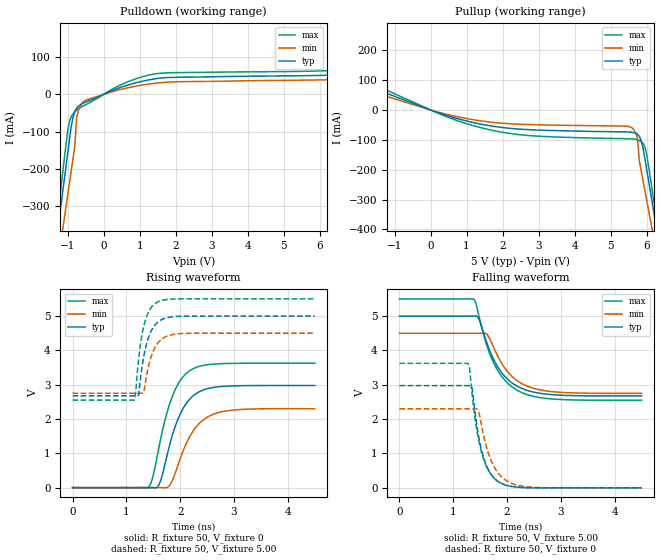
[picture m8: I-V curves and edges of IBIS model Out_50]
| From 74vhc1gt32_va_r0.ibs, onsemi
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|//////////////////////////////////////////////////////////////////////////////
|//////////////////////////////////////////////////////////////////////////////
[Model] Out_50
Model_type Output
Polarity Non-Inverting
Vmeas = 2.50
Vref = 5.00
Rref = 1k
Cref = 15pF
|  variable   typ   min   max
C_comp   3.9pF   3.9pF   3.9pF
|//////////////////////////////////////////////////////////////////////////////
[Temperature Range]   25   125   -55
|//////////////////////////////////////////////////////////////////////////////
[Voltage Range]   5.00V   4.50V   5.50V
|//////////////////////////////////////////////////////////////////////////////
[Pulldown Reference]   0V   0V   0V
|//////////////////////////////////////////////////////////////////////////////
[Pullup Reference]   5.00V   4.50V   5.50V
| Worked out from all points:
|   slope of the pulldown table from 0 to 0.75 V, typ, clamps not added: 27.5 ohm
|   slope of the pullup table from 0 to 0.75 V, typ, clamps not added: 25.7 ohm
|   falling waveform, R_fixture 50, V_fixture 5.00: 20-80 % time 466ps typ, 472ps min, 463ps max; typ from 5 V to 2.67 V
|   falling waveform, R_fixture 50, V_fixture 0: 20-80 % time 239ps typ, 298ps min, 250ps max; typ from 2.98 V to 0 V
|   rising waveform, R_fixture 50, V_fixture 0: 20-80 % time 378ps typ, 421ps min, 372ps max; typ from 0 V to 2.98 V
|   rising waveform, R_fixture 50, V_fixture 5.00: 20-80 % time 192ps typ, 200ps min, 168ps max; typ from 2.67 V to 5 V
|//////////////////////////////////////////////////////////////////////////////
[Pulldown]
|   Voltage   I(typ)   I(min)   I(max)
-5V       -3.203A    -2.93A     -3.469A
-1.4V     -459.9mA   -538mA     -431.9mA
-1.25V    -347.3mA   -438.3mA   -305.4mA
-1.15V    -272.2mA   -371.8mA   -221.3mA
-950mV    -121.9mA   -238.6mA   -72.82mA
-850mV    -61mA      -171.9mA   -52.46mA
-750mV    -36.79mA   -62.89mA   -42.39mA
-700mV    -31.75mA   -43.7mA    -38.5mA
125mV     5.571mA    3.909mA    7.607mA
1.5V      42.83mA    30.68mA    56.15mA
8V        63.99mA    47.99mA    80.81mA
10V       113.3mA    83.22mA    177.5mA
|//////////////////////////////////////////////////////////////////////////////
[Pullup]
|   Voltage   I(typ)   I(min)   I(max)
-5V       205mA      169.6mA    275.2mA
-3.8V     161.9mA    134.7mA    191.7mA
1.15V     -41.19mA   -31.93mA   -51.29mA
5.55V     -74.1mA    -57.09mA   -96.6mA
5.75V     -81.39mA   -96.38mA   -99.99mA
5.8V      -88.37mA   -170.9mA   -102.6mA
5.85V     -102.5mA   -203.1mA   -106mA
6V        -196.5mA   -299.9mA   -146.2mA
6.15V     -305mA     -396.6mA   -263.3mA
6.25V     -377.3mA   -461.2mA   -343.4mA
6.4V      -485.9mA   -558mA     -463.7mA
10V       -3.241A    -3.004A    -3.527A
|//////////////////////////////////////////////////////////////////////////////
|//////////////////////////////////////////////////////////////////////////////
[Ramp]
|  variable   typ   min   max
dV/dt_f   1.395E+00/4.500E-10  1.050E+00/4.750E-10  1.770E+00/4.750E-10
dV/dt_r   1.785E+00/3.750E-10  1.380E+00/4.250E-10  2.175E+00/3.750E-10
R_load = 50
|/////////////////////////////////////////////////////////////////////////////
[Falling Waveform]
R_fixture = 50
V_fixture = 5.00
V_fixture_min = 4.50
V_fixture_max = 5.50
C_fixture = 0p
|   time   V(typ)   V(min)   V(max)
0s        5V         4.5V       5.5V
1.375ns   5.001V     4.5V       5.5V
1.425ns   5.001V     4.5V       5.343V
1.475ns   4.921V     4.5V       5.016V
1.625ns   4.214V     4.472V     4.138V
1.775ns   3.661V     4V         3.561V
2ns       3.175V     3.398V     3.064V
2.275ns   2.893V     3.032V     2.773V
2.9ns     2.706V     2.792V     2.58V
4.5ns     2.675V     2.75V      2.55V
|//////////////////////////////////////////////////////////////////////////////
[Falling Waveform]
R_fixture = 50
V_fixture = 0
C_fixture = 0p
|   time   V(typ)   V(min)   V(max)
0s        2.975V     2.3V       3.625V
1.275ns   2.975V     2.3V       3.624V
1.3ns     2.975V     2.3V       3.522V
1.35ns    2.905V     2.3V       2.73V
1.45ns    1.698V     2.287V     1.569V
1.525ns   1.1V       1.82V      1.036V
1.675ns   460.6mV    907.4mV    450mV
1.875ns   141.5mV    356.1mV    146.3mV
2.45ns    1.172mV    20.8mV     1.891mV
4.5ns     0V         0V         0V
|//////////////////////////////////////////////////////////////////////////////
[Rising Waveform]
R_fixture = 50
V_fixture = 0
C_fixture = 0p
|   time   V(typ)   V(min)   V(max)
0s        0V         0V         0V
1.425ns   445.8uV    69.84uV    39.66mV
1.5ns     -2.61mV    73.52uV    367.8mV
1.625ns   153.4mV    1.202mV    1.332V
1.85ns    1.504V     194.7mV    2.643V
2.025ns   2.223V     950.9mV    3.175V
2.225ns   2.653V     1.613V     3.451V
2.45ns    2.856V     1.998V     3.567V
2.8ns     2.951V     2.22V      3.615V
4.5ns     2.975V     2.3V       3.625V
|//////////////////////////////////////////////////////////////////////////////
[Rising Waveform]
R_fixture = 50
V_fixture = 5.00
V_fixture_min = 4.50
V_fixture_max = 5.50
C_fixture = 0p
|   time   V(typ)   V(min)   V(max)
0s        2.675V     2.75V      2.55V
1.15ns    2.675V     2.75V      2.55V
1.175ns   2.675V     2.75V      2.803V
1.225ns   2.692V     2.75V      3.716V
1.275ns   3.34V      2.75V      4.317V
1.325ns   3.842V     2.788V     4.716V
1.45ns    4.529V     3.765V     5.223V
1.6ns     4.843V     4.241V     5.423V
2.025ns   4.995V     4.489V     5.5V
4.5ns     5V         4.5V       5.5V
